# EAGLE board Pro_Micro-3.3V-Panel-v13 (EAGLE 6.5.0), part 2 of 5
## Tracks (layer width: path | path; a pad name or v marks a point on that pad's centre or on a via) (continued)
A16
  Top 0.203: U6.37 56.7,23.8 58.35,23.8 58.7,23.45 58.7,22.86 59.94,21.62 JP9.7
A17
  Top 0.203: U6.36 56.96,23.38 58.04,23.38 58.21,23.2 58.21,22.8 58.7,22.3 58.7,19.53 JP9.8
A20
  Top 0.203: 74.4,24.62 74.41,24.62 | 73.32,23.54 74.41,24.62 | 74.41,24.62 76.94,24.62 JP13.5
A21
  Top 0.203: U8.38 74.7,24.22 77.38,24.22 JP13.6
A22
  Top 0.203: U8.37 74.98,23.8 76.63,23.8 76.99,23.45 76.99,22.86 78.23,21.62 JP13.7
A23
  Top 0.203: U8.36 75.25,23.38 76.33,23.38 76.5,23.2 76.5,22.8 76.99,22.3 76.99,19.53 JP13.8
A26
  Top 0.203: 92.69,24.62 92.7,24.62 | 91.61,23.54 92.7,24.62 | 92.7,24.62 95.23,24.62 JP17.5
A27
  Top 0.203: U10.38 92.99,24.22 95.67,24.22 JP17.6
A28
  Top 0.203: U10.37 93.27,23.8 94.92,23.8 95.28,23.45 95.28,22.86 96.52,21.62 JP17.7
A29
  Top 0.203: U10.36 93.54,23.38 94.62,23.38 94.79,23.2 94.79,22.8 95.28,22.3 95.28,19.53 JP17.8
A32
  Top 0.203: 110.98,24.62 | 109.9,23.54 110.98,24.62 | 110.98,24.62 113.52,24.62 JP21.5
A33
  Top 0.203: U12.38 111.28,24.22 113.95,24.22 JP21.6
A34
  Top 0.203: U12.37 111.56,23.8 113.21,23.8 113.57,23.45 113.57,22.86 114.81,21.62 JP21.7
A35
  Top 0.203: U12.36 111.83,23.38 112.91,23.38 113.08,23.2 113.08,22.8 113.57,22.3 113.57,19.53 JP21.8
A38
  Top 0.203: 19.54,61.45 19.55,61.45 | 18.46,60.37 19.55,61.45 | 19.55,61.45 22.08,61.45 JP25.5
A39
  Top 0.203: U14.38 19.84,61.05 22.52,61.05 JP25.6
A40
  Top 0.203: U14.37 20.12,60.63 21.77,60.63 22.13,60.28 22.13,59.7 23.37,58.45 JP25.7
A41
  Top 0.203: U14.36 20.39,60.21 21.47,60.21 21.64,60.03 21.64,59.63 22.13,59.13 22.13,56.36 JP25.8
A44
  Top 0.203: 37.83,61.45 | 36.74,60.37 37.83,61.45 | 37.83,61.45 40.37,61.45 41.65,62.74 JP29.5
A45
  Top 0.203: U16.38 38.13,61.05 40.8,61.05 JP29.6
A46
  Top 0.203: U16.37 38.41,60.63 40.06,60.63 40.41,60.28 40.41,59.7 41.66,58.45 JP29.7
A47
  Top 0.203: U16.36 38.67,60.21 39.75,60.21 39.92,60.03 39.92,59.63 40.42,59.13 40.42,56.36 JP29.8
A50
  Top 0.203: 56.11,61.45 56.12,61.45 | 55.03,60.37 56.12,61.45 | 56.12,61.45 58.65,61.45 JP33.5
A51
  Top 0.203: U18.38 56.41,61.05 59.09,61.05 JP33.6
A52
  Top 0.203: U18.37 56.7,60.63 58.35,60.63 58.7,60.28 58.7,59.7 59.94,58.45 JP33.7
A53
  Top 0.203: U18.36 56.96,60.21 58.04,60.21 58.21,60.03 58.21,59.63 58.7,59.13 58.7,56.36 JP33.8
A56
  Top 0.203: 74.4,61.45 74.41,61.45 | 73.32,60.37 74.41,61.45 | 74.41,61.45 76.94,61.45 JP37.5
A57
  Top 0.203: U20.38 74.7,61.05 77.38,61.05 JP37.6
A58
  Top 0.203: U20.37 74.98,60.63 76.63,60.63 76.99,60.28 76.99,59.7 78.23,58.45 JP37.7
A59
  Top 0.203: U20.36 75.25,60.21 76.33,60.21 76.5,60.03 76.5,59.63 76.99,59.13 76.99,56.36 JP37.8
A62
  Top 0.203: 92.69,61.45 92.7,61.45 | 91.61,60.37 92.7,61.45 | 92.7,61.45 95.23,61.45 JP41.5
A63
  Top 0.203: U22.38 92.99,61.05 95.67,61.05 JP41.6
A64
  Top 0.203: U22.37 93.27,60.63 94.92,60.63 95.28,60.28 95.28,59.7 96.52,58.45 JP41.7
A65
  Top 0.203: U22.36 93.54,60.21 94.62,60.21 94.79,60.03 94.79,59.63 95.28,59.13 95.28,56.36 JP41.8
A68
  Top 0.203: 110.98,61.45 | 109.9,60.37 110.98,61.45 | 110.98,61.45 113.52,61.45 JP45.5
A69
  Top 0.203: U24.38 111.28,61.05 113.95,61.05 JP45.6
A70
  Top 0.203: U24.37 111.56,60.63 113.21,60.63 113.57,60.28 113.57,59.7 114.81,58.45 JP45.7
A71
  Top 0.203: U24.36 111.83,60.21 112.91,60.21 113.08,60.03 113.08,59.63 113.57,59.13 113.57,56.36 JP45.8
A74
  Top 0.203: 19.54,98.28 19.55,98.28 | 18.46,97.2 19.55,98.28 | 19.55,98.28 22.08,98.28 JP49.5
A75
  Top 0.203: U26.38 19.84,97.88 22.52,97.88 JP49.6
A76
  Top 0.203: U26.37 20.12,97.47 21.77,97.47 22.13,97.11 22.13,96.53 23.37,95.28 JP49.7
A77
  Top 0.203: U26.36 20.39,97.04 21.47,97.04 21.64,96.86 21.64,96.46 22.13,95.96 22.13,93.19 JP49.8
A80
  Top 0.203: 37.83,98.28 | 36.74,97.2 37.83,98.28 | 37.83,98.28 40.37,98.28 41.65,99.57 JP53.5
A81
  Top 0.203: U28.38 38.13,97.88 40.8,97.88 JP53.6
A82
  Top 0.203: U28.37 38.41,97.47 40.06,97.47 40.41,97.11 40.41,96.53 41.66,95.28 JP53.7
A83
  Top 0.203: U28.36 38.67,97.04 39.75,97.04 39.92,96.86 39.92,96.46 40.42,95.96 40.42,93.19 JP53.8
A86
  Top 0.203: 56.11,98.28 56.12,98.28 | 55.03,97.2 56.12,98.28 | 56.12,98.28 58.65,98.28 JP57.5
A87
  Top 0.203: U30.38 56.41,97.88 59.09,97.88 JP57.6
A88
  Top 0.203: U30.37 56.7,97.47 58.35,97.47 58.7,97.11 58.7,96.53 59.94,95.28 JP57.7
A89
  Top 0.203: U30.36 56.96,97.04 58.04,97.04 58.21,96.86 58.21,96.46 58.7,95.96 58.7,93.19 JP57.8
A92
  Top 0.203: 74.4,98.28 74.41,98.28 | 73.32,97.2 74.41,98.28 | 74.41,98.28 76.94,98.28 JP61.5
A93
  Top 0.203: U32.38 74.7,97.88 77.38,97.88 JP61.6
A94
  Top 0.203: U32.37 74.98,97.47 76.63,97.47 76.99,97.11 76.99,96.53 78.23,95.28 JP61.7
A95
  Top 0.203: U32.36 75.25,97.04 76.33,97.04 76.5,96.86 76.5,96.46 76.99,95.96 76.99,93.19 JP61.8
A98
  Top 0.203: 92.69,98.28 92.7,98.28 | 91.61,97.2 92.7,98.28 | 92.7,98.28 95.23,98.28 JP65.5
A99
  Top 0.203: U34.38 92.99,97.88 95.67,97.88 JP65.6
A100
  Top 0.203: U34.37 93.27,97.47 94.92,97.47 95.28,97.11 95.28,96.53 96.52,95.28 JP65.7
A101
  Top 0.203: U34.36 93.54,97.04 94.62,97.04 94.79,96.86 94.79,96.46 95.28,95.96 95.28,93.19 JP65.8
A104
  Top 0.203: 110.98,98.28 | 109.9,97.2 110.98,98.28 | 110.98,98.28 113.52,98.28 JP69.5
A105
  Top 0.203: U36.38 111.28,97.88 113.95,97.88 JP69.6
A106
  Top 0.203: U36.37 111.56,97.47 113.21,97.47 113.57,97.11 113.57,96.53 114.81,95.28 JP69.7
A107
  Top 0.203: U36.36 111.83,97.04 112.91,97.04 113.08,96.86 113.08,96.46 113.57,95.96 113.57,93.19 JP69.8
AREF
  Top 0.203: 17.41,24.58 18.24,25.41 C1.2
AREF1
  Top 0.203: 35.7,24.58 36.53,25.41 C11.2
AREF2
  Top 0.203: 53.99,24.58 54.82,25.41 C22.2
AREF3
  Top 0.203: 72.27,24.58 73.11,25.41 C31.2
AREF4
  Top 0.203: 90.56,24.58 91.4,25.41 C40.2
AREF5
  Top 0.203: 108.85,24.58 109.68,25.41 C49.2
AREF6
  Top 0.203: 17.41,61.41 18.24,62.24 C58.2
AREF7
  Top 0.203: 35.7,61.41 36.53,62.24 C67.2
AREF8
  Top 0.203: 53.99,61.41 54.82,62.24 C76.2
AREF9
  Top 0.203: 72.27,61.41 73.11,62.24 C85.2
AREF10
  Top 0.203: 90.56,61.41 91.4,62.24 C94.2
AREF11
  Top 0.203: 108.85,61.41 109.68,62.24 C103.2
AREF12
  Top 0.203: 17.41,98.24 18.24,99.08 C112.2
AREF13
  Top 0.203: 35.7,98.24 36.53,99.08 C121.2
AREF14
  Top 0.203: 53.99,98.24 54.82,99.08 C130.2
AREF15
  Top 0.203: 72.27,98.24 73.11,99.08 C139.2
AREF16
  Top 0.203: 90.56,98.24 91.4,99.08 C148.2
AREF17
  Top 0.203: 108.85,98.24 109.68,99.08 C157.2
D1  (via drill 0.25)
  Top 0.203: 37.09,18.47 38.4,17.16 39.23,17.16 39.98,16.41 39.98,9.35 40.26,9.06 v40.3,9.06
  Bottom 0.203: JP4.1 27.18,7.37 39.9,7.37 40.3,7.77 v40.3,9.06
D2  (via drill 0.25)
  Top 0.203: 13.74,17.42 13.56,17.25 13.56,16.57 v13.31,16.32
  Bottom 0.203: v13.31,16.32 14.48,17.49 14.48,18.29 11.68,21.08 11.68,23.55 11.09,24.14 10.13,24.14 9.79,24.49 9.79,27.08 10.3,27.58 11.01,27.58 11.68,28.25 11.68,30.62 11.68,30.63 11.11,31.21 9.91,31.21 9.41,30.7 9.41,27.9 8.13,26.62 JP7.8
D3  (via drill 0.25)
  Top 0.203: 13.39,17.77 12.88,17.26 v12.85,17.26
  Bottom 0.203: JP7.7 9.4,22.1 9.4,20.32 9.91,19.81 9.91,18.41 11.06,17.26 v12.85,17.26
D4  (via drill 0.25)
  Top 0.203: 17.41,17.07 18.46,16.03 v18.46,15.62
  Bottom 0.203: JP7.6 9.4,19.56 9.4,17.58 9.78,17.2 9.78,14.81 10.27,14.31 10.27,12.12 10.75,11.65 15.79,11.65 17.44,13.3 17.44,13.96 18.46,14.98 v18.46,15.62
D5  (via drill 0.25)
  Top 0.203: 19.5,19.17 20.13,18.53 v20.49,18.53
  Bottom 0.203: JP7.5 9.4,17.02 9.4,15.24 9.36,15.2 9.36,14.62 9.85,14.12 9.85,11.93 10.62,11.16 15.91,11.16 17.86,13.1 17.86,13.72 17.87,13.72 18.57,14.41 19.11,14.41 19.72,15.02 19.72,15.55 18.97,16.3 17.99,16.3 17.7,16.59 17.7,17.42 18.27,17.99 19.94,17.99 v20.49,18.53
D6  (via drill 0.25)
  Top 0.203: v18.41,17.14 18.41,17.45 v18.41,17.14 | U3.27 18.41,17.46 v18.41,17.14
  Bottom 0.203: v18.41,17.14 18.86,17.14 20.23,15.78 20.23,14.88 19.35,14.01 18.73,14.01 18.27,13.55 18.27,12.88 16.03,10.63 10.39,10.63 9.37,11.66 9.37,13.93 8.13,15.17 JP7.4
D7  (via drill 0.25)
  Top 0.203: JP7.3 9.4,14.48 9.4,20.14 v10.09,20.83 | v10.56,30.44 10.56,30.4 10.77,30.18 10.77,29.34 11.03,29.07 12.8,29.07 13.05,29.32 13.52,29.32 13.95,28.89 13.95,28.3 13.7,28.05 13.7,27.37 13.89,27.19 15.57,27.19 15.57,27.17 15.95,26.79 16.58,26.79 16.68,26.68 16.68,25.93 16.1,25.34 15.4,25.34 15.1,25.64 14.93,25.64 14.78,25.5 14.78,25.28 U3.1 14.79,25.28
  Bottom 0.203: v10.56,30.44 10.52,30.44 9.86,29.78 9.86,27.75 9.4,27.29 9.4,22.99 10.09,22.3 v10.09,20.83
D8  (via drill 0.25)
  Top 0.203: U3.28 19.84,16.74 20.66,16.74 21.23,16.16 21.23,9.53 21.25,9.51 v21.25,8.12
  Bottom 0.203: JP7.2 11,7.8 20.93,7.8 v21.25,8.12
D9  (via drill 0.25)
  Top 0.203: 18.8,18.47 20.12,17.16 20.94,17.16 21.69,16.41 21.69,9.35 21.97,9.06 v22.02,9.06
  Bottom 0.203: JP7.1 8.89,7.37 21.61,7.37 22.02,7.77 v22.02,9.06
D10
  Top 0.203: JP6.12 23.37,8.81 22.12,10.06 22.12,16.56 21.1,17.58 20.39,17.58 U3.30
D14  (via drill 0.25)
  Top 0.203: R4.1 9.65,9.56 9.65,11.68 9.81,11.84 9.81,18.19 v10.57,18.96 | 12.35,22.83 11.81,23.37 v10.92,23.37
  Bottom 0.203: v10.92,23.37 10.92,19.31 v10.57,18.96
D15  (via drill 0.25)
  Top 0.203: U4.28 38.13,16.74 38.95,16.74 39.52,16.16 39.52,9.53 39.53,9.51 v39.53,8.12
  Bottom 0.203: JP4.2 29.29,7.8 39.22,7.8 v39.53,8.12
D16  (via drill 0.25)
  Top 0.203: 32.02,17.42 31.85,17.25 31.85,16.57 v31.59,16.32
  Bottom 0.203: v31.59,16.32 32.77,17.49 32.77,18.29 29.97,21.08 29.97,23.55 29.38,24.14 28.42,24.14 28.08,24.49 28.08,27.08 28.59,27.58 29.3,27.58 29.97,28.25 29.97,30.62 29.97,30.63 29.39,31.21 28.2,31.21 27.7,30.7 27.7,27.9 26.42,26.62 JP4.8
D17  (via drill 0.25)
  Top 0.203: 31.68,17.77 31.17,17.26 v31.14,17.26
  Bottom 0.203: JP4.7 27.69,22.1 27.69,20.32 28.19,19.81 28.19,18.41 29.34,17.26 v31.14,17.26
D18  (via drill 0.25)
  Top 0.203: 35.7,17.07 36.74,16.03 v36.74,15.62
  Bottom 0.203: JP4.6 27.69,19.56 27.69,17.58 28.07,17.2 28.07,14.81 28.56,14.31 28.56,12.12 29.04,11.65 34.07,11.65 35.73,13.3 35.73,13.96 36.74,14.98 v36.74,15.62
D19  (via drill 0.25)
  Top 0.203: 37.79,19.17 38.42,18.53 v38.78,18.53
  Bottom 0.203: JP4.5 27.69,17.02 27.69,15.24 27.64,15.2 27.64,14.62 28.14,14.12 28.14,11.93 28.91,11.16 34.2,11.16 36.14,13.1 36.14,13.72 36.16,13.72 36.85,14.41 37.4,14.41 38.01,15.02 38.01,15.55 37.26,16.3 36.28,16.3 35.99,16.59 35.99,17.42 36.56,17.99 38.23,17.99 v38.78,18.53
D20  (via drill 0.25)
  Top 0.203: v36.7,17.14 36.7,17.45 v36.7,17.14 | U4.27 36.7,17.46 v36.7,17.14
  Bottom 0.203: v36.7,17.14 37.15,17.14 38.52,15.78 38.52,14.88 37.64,14.01 37.02,14.01 36.56,13.55 36.56,12.88 34.31,10.63 28.68,10.63 27.66,11.66 27.66,13.93 26.42,15.17 JP4.4
D21  (via drill 0.25)
  Top 0.203: JP4.3 27.69,14.48 27.69,20.14 v28.38,20.83 | v28.84,30.44 28.84,30.4 29.06,30.18 29.06,29.34 29.32,29.07 31.09,29.07 31.34,29.32 31.81,29.32 32.23,28.89 32.23,28.3 31.99,28.05 31.99,27.37 32.17,27.19 33.86,27.19 33.86,27.17 34.24,26.79 34.86,26.79 34.97,26.68 34.97,25.93 34.38,25.34 33.69,25.34 33.39,25.64 33.21,25.64 33.07,25.5 33.07,25.28 U4.1 33.07,25.28
  Bottom 0.203: v28.84,30.44 28.81,30.44 28.14,29.78 28.14,27.75 27.69,27.29 27.69,22.99 28.38,22.3 v28.38,20.83
D22
  Top 0.203: JP3.12 41.66,8.81 40.41,10.06 40.41,16.56 39.38,17.58 38.67,17.58 U4.30
D26  (via drill 0.25)
  Top 0.203: R9.1 27.94,9.56 27.94,11.68 28.09,11.84 28.09,18.19 v28.86,18.96 | 30.64,22.83 30.1,23.37 v29.21,23.37
  Bottom 0.203: v29.21,23.37 29.21,19.31 v28.86,18.96
D27  (via drill 0.25)
  Top 0.203: 55.38,18.47 56.69,17.16 57.52,17.16 58.27,16.41 58.27,9.35 58.55,9.06 v58.59,9.06
  Bottom 0.203: JP10.1 45.47,7.37 58.19,7.37 58.59,7.77 v58.59,9.06
D28  (via drill 0.25)
  Top 0.203: U6.28 56.42,16.74 57.24,16.74 57.81,16.16 57.81,9.53 57.82,9.51 v57.82,8.12
  Bottom 0.203: JP10.2 47.57,7.8 57.5,7.8 v57.82,8.12
D29  (via drill 0.25)
  Top 0.203: 50.31,17.42 50.14,17.25 50.14,16.57 v49.88,16.32
  Bottom 0.203: v49.88,16.32 51.05,17.49 51.05,18.29 48.26,21.08 48.26,23.55 47.67,24.14 46.71,24.14 46.37,24.49 46.37,27.08 46.88,27.58 47.59,27.58 48.26,28.25 48.26,30.62 48.26,30.63 47.68,31.21 46.49,31.21 45.99,30.7 45.99,27.9 44.7,26.62 JP10.8
D30  (via drill 0.25)
  Top 0.203: 49.97,17.77 49.96,17.77 49.46,17.26 v49.42,17.26
  Bottom 0.203: JP10.7 45.97,22.1 45.97,20.32 46.48,19.81 46.48,18.41 47.63,17.26 v49.42,17.26
D31  (via drill 0.25)
  Top 0.203: 53.99,17.07 55.03,16.03 v55.03,15.62
  Bottom 0.203: JP10.6 45.97,19.56 45.97,17.58 46.35,17.2 46.35,14.81 46.85,14.31 46.85,12.12 47.33,11.65 52.36,11.65 54.02,13.3 54.02,13.96 55.03,14.98 v55.03,15.62
D32  (via drill 0.25)
  Top 0.203: 56.08,19.17 56.71,18.53 v57.06,18.53
  Bottom 0.203: JP10.5 45.97,17.02 45.97,15.24 45.93,15.2 45.93,14.62 46.43,14.12 46.43,11.93 47.19,11.16 52.49,11.16 54.43,13.1 54.43,13.72 54.45,13.72 55.14,14.41 55.68,14.41 56.29,15.02 56.29,15.55 55.55,16.3 54.56,16.3 54.28,16.59 54.28,17.42 54.85,17.99 56.52,17.99 v57.06,18.53
D33  (via drill 0.25)
  Top 0.203: v54.99,17.14 54.99,17.45 v54.99,17.14 | U6.27 54.99,17.46 v54.99,17.14
  Bottom 0.203: v54.99,17.14 55.44,17.14 56.81,15.78 56.81,14.88 55.93,14.01 55.31,14.01 54.85,13.55 54.85,12.88 52.6,10.63 46.97,10.63 45.95,11.66 45.95,13.93 44.7,15.17 JP10.4
D34  (via drill 0.25)
  Top 0.203: JP10.3 45.97,14.48 45.97,20.14 v46.66,20.83 | v47.13,30.44 47.13,30.4 47.35,30.18 47.35,29.34 47.61,29.07 49.38,29.07 49.63,29.32 50.09,29.32 50.52,28.89 50.52,28.3 50.28,28.05 50.28,27.37 50.46,27.19 52.15,27.19 52.15,27.17 52.53,26.79 53.15,26.79 53.25,26.68 53.25,25.93 52.67,25.34 51.98,25.34 51.68,25.64 51.5,25.64 51.35,25.5 51.35,25.28 U6.1 51.36,25.28
  Bottom 0.203: v47.13,30.44 47.1,30.44 46.43,29.78 46.43,27.75 45.97,27.29 45.97,22.99 46.66,22.3 v46.66,20.83
D35
  Top 0.203: JP9.12 59.94,8.81 58.7,10.06 58.7,16.56 57.67,17.58 56.96,17.58 U6.30
D39  (via drill 0.25)
  Top 0.203: R16.1 46.23,9.56 46.23,11.68 46.38,11.84 46.38,18.19 v47.15,18.96 | 48.93,22.83 48.39,23.37 v47.5,23.37
  Bottom 0.203: v47.5,23.37 47.5,19.31 v47.15,18.96
D40  (via drill 0.25)
  Top 0.203: 73.67,18.47 74.98,17.16 75.81,17.16 76.56,16.41 76.56,9.35 76.84,9.06 v76.88,9.06
  Bottom 0.203: JP14.1 63.75,7.37 76.48,7.37 76.88,7.77 v76.88,9.06
D41  (via drill 0.25)
  Top 0.203: U8.28 74.7,16.74 75.53,16.74 76.1,16.16 76.1,9.53 76.11,9.51 v76.11,8.12
  Bottom 0.203: JP14.2 65.86,7.8 75.79,7.8 v76.11,8.12
D42  (via drill 0.25)
  Top 0.203: 68.6,17.42 68.43,17.25 68.43,16.57 v68.17,16.32
  Bottom 0.203: v68.17,16.32 69.34,17.49 69.34,18.29 66.55,21.08 66.55,23.55 65.96,24.14 65,24.14 64.66,24.49 64.66,27.08 65.16,27.58 65.88,27.58 66.55,28.25 66.55,30.62 66.55,30.63 65.97,31.21 64.78,31.21 64.28,30.7 64.28,27.9 62.99,26.62 JP14.8
D43  (via drill 0.25)
  Top 0.203: 68.25,17.77 67.74,17.26 v67.71,17.26
  Bottom 0.203: JP14.7 64.26,22.1 64.26,20.32 64.77,19.81 64.77,18.41 65.92,17.26 v67.71,17.26
D44  (via drill 0.25)
  Top 0.203: 72.27,17.07 73.32,16.03 v73.32,15.62
  Bottom 0.203: JP14.6 64.26,19.56 64.26,17.58 64.64,17.2 64.64,14.81 65.14,14.31 65.14,12.12 65.61,11.65 70.65,11.65 72.31,13.3 72.31,13.96 73.32,14.98 v73.32,15.62
D45  (via drill 0.25)
  Top 0.203: 74.37,19.17 75,18.53 v75.35,18.53
  Bottom 0.203: JP14.5 64.26,17.02 64.26,15.24 64.22,15.2 64.22,14.62 64.72,14.12 64.72,11.93 65.48,11.16 70.78,11.16 72.72,13.1 72.72,13.72 72.73,13.72 73.43,14.41 73.97,14.41 74.58,15.02 74.58,15.55 73.83,16.3 72.85,16.3 72.57,16.59 72.57,17.42 73.13,17.99 74.81,17.99 v75.35,18.53
D46  (via drill 0.25)
  Top 0.203: v73.28,17.14 73.28,17.45 v73.28,17.14 | U8.27 73.28,17.46 v73.28,17.14
  Bottom 0.203: v73.28,17.14 73.73,17.14 75.09,15.78 75.09,14.88 74.22,14.01 73.59,14.01 73.13,13.55 73.13,12.88 70.89,10.63 65.25,10.63 64.23,11.66 64.23,13.93 62.99,15.17 JP14.4
D47  (via drill 0.25)
  Top 0.203: JP14.3 64.26,14.48 64.26,20.14 v64.95,20.83 | v65.42,30.44 65.42,30.4 65.63,30.18 65.63,29.34 65.89,29.07 67.67,29.07 67.92,29.32 68.38,29.32 68.81,28.89 68.81,28.3 68.57,28.05 68.57,27.37 68.75,27.19 70.44,27.19 70.44,27.17 70.82,26.79 71.44,26.79 71.54,26.68 71.54,25.93 70.96,25.34 70.27,25.34 69.97,25.64 69.79,25.64 69.64,25.5 69.64,25.28 U8.1 69.65,25.28
  Bottom 0.203: v65.42,30.44 65.39,30.44 64.72,29.78 64.72,27.75 64.26,27.29 64.26,22.99 64.95,22.3 v64.95,20.83
D48
  Top 0.203: JP13.12 78.23,8.81 76.99,10.06 76.99,16.56 75.96,17.58 75.25,17.58 U8.30
D52  (via drill 0.25)
  Top 0.203: R22.1 64.52,9.56 64.52,11.68 64.67,11.84 64.67,18.19 v65.44,18.96 | 67.22,22.83 66.68,23.37 v65.79,23.37
  Bottom 0.203: v65.79,23.37 65.79,19.31 v65.44,18.96
D53  (via drill 0.25)
  Top 0.203: 91.96,18.47 93.27,17.16 94.09,17.16 94.84,16.41 94.84,9.35 95.13,9.06 v95.17,9.06
  Bottom 0.203: JP18.1 82.04,7.37 94.77,7.37 95.17,7.77 v95.17,9.06
D54  (via drill 0.25)
  Top 0.203: U10.28 92.99,16.74 93.81,16.74 94.39,16.16 94.39,9.53 94.4,9.51 v94.4,8.12
  Bottom 0.203: JP18.2 84.15,7.8 94.08,7.8 v94.4,8.12
D55  (via drill 0.25)
  Top 0.203: 86.89,17.42 86.72,17.25 86.72,16.57 v86.46,16.32
  Bottom 0.203: v86.46,16.32 87.63,17.49 87.63,18.29 84.84,21.08 84.84,23.55 84.24,24.14 83.29,24.14 82.94,24.49 82.94,27.08 83.45,27.58 84.16,27.58 84.83,28.25 84.83,30.62 84.84,30.63 84.26,31.21 83.07,31.21 82.56,30.7 82.56,27.9 81.28,26.62 JP18.8
D56  (via drill 0.25)
  Top 0.203: 86.54,17.77 86.03,17.26 v86,17.26
  Bottom 0.203: JP18.7 82.55,22.1 82.55,20.32 83.06,19.81 83.06,18.41 84.21,17.26 v86,17.26
D57  (via drill 0.25)
  Top 0.203: 90.56,17.07 91.61,16.03 v91.61,15.62
  Bottom 0.203: JP18.6 82.55,19.56 82.55,17.58 82.93,17.2 82.93,14.81 83.43,14.31 83.43,12.12 83.9,11.65 88.94,11.65 90.59,13.3 90.59,13.96 91.61,14.98 v91.61,15.62
D58  (via drill 0.25)
  Top 0.203: 92.65,19.17 93.28,18.53 v93.64,18.53
  Bottom 0.203: JP18.5 82.55,17.02 82.55,15.24 82.51,15.2 82.51,14.62 83,14.12 83,11.93 83.77,11.16 89.06,11.16 91.01,13.1 91.01,13.72 91.02,13.72 91.72,14.41 92.26,14.41 92.87,15.02 92.87,15.55 92.12,16.3 91.14,16.3 90.86,16.59 90.86,17.42 91.42,17.99 93.1,17.99 v93.64,18.53
D59  (via drill 0.25)
  Top 0.203: v91.57,17.14 91.57,17.45 v91.57,17.14 | U10.27 91.57,17.46 v91.57,17.14
  Bottom 0.203: v91.57,17.14 92.02,17.14 93.38,15.78 93.38,14.88 92.5,14.01 91.88,14.01 91.42,13.55 91.42,12.88 89.18,10.63 83.54,10.63 82.52,11.66 82.52,13.93 81.28,15.17 JP18.4
D60  (via drill 0.25)
  Top 0.203: JP18.3 82.55,14.48 82.55,20.14 v83.24,20.83 | v83.71,30.44 83.71,30.4 83.92,30.18 83.92,29.34 84.18,29.07 85.96,29.07 86.2,29.32 86.67,29.32 87.1,28.89 87.1,28.3 86.86,28.05 86.86,27.37 87.04,27.19 88.72,27.19 88.72,27.17 89.11,26.79 89.73,26.79 89.83,26.68 89.83,25.93 89.25,25.34 88.56,25.34 88.25,25.64 88.08,25.64 87.93,25.5 87.93,25.28 U10.1 87.94,25.28
  Bottom 0.203: v83.71,30.44 83.67,30.44 83.01,29.78 83.01,27.75 82.55,27.29 82.55,22.99 83.24,22.3 v83.24,20.83
D61
  Top 0.203: JP17.12 96.52,8.81 95.28,10.06 95.28,16.56 94.25,17.58 93.54,17.58 U10.30
D65  (via drill 0.25)
  Top 0.203: R28.1 82.8,9.56 82.8,11.68 82.96,11.84 82.96,18.19 v83.73,18.96 | 85.51,22.83 84.97,23.37 v84.07,23.37
  Bottom 0.203: v84.07,23.37 84.07,19.31 v83.73,18.96
D66  (via drill 0.25)
  Top 0.203: 110.24,18.47 111.56,17.16 112.38,17.16 113.13,16.41 113.13,9.35 113.41,9.06 v113.46,9.06
  Bottom 0.203: JP22.1 100.33,7.37 113.06,7.37 113.46,7.77 v113.46,9.06
D67  (via drill 0.25)
  Top 0.203: U12.28 111.28,16.74 112.1,16.74 112.67,16.16 112.67,9.53 112.69,9.51 v112.69,8.12
  Bottom 0.203: JP22.2 102.44,7.8 112.37,7.8 v112.69,8.12
D68  (via drill 0.25)
  Top 0.203: 105.18,17.42 105,17.25 105,16.57 v104.75,16.32
  Bottom 0.203: v104.75,16.32 105.92,17.49 105.92,18.29 103.12,21.08 103.12,23.55 102.53,24.14 101.58,24.14 101.23,24.49 101.23,27.08 101.74,27.58 102.45,27.58 103.12,28.25 103.12,30.62 103.12,30.63 102.55,31.21 101.35,31.21 100.85,30.7 100.85,27.9 99.57,26.62 JP22.8
D69  (via drill 0.25)
  Top 0.203: 104.83,17.77 104.32,17.26 v104.29,17.26
  Bottom 0.203: JP22.7 100.84,22.1 100.84,20.32 101.35,19.81 101.35,18.41 102.5,17.26 v104.29,17.26
D70  (via drill 0.25)
  Top 0.203: 108.85,17.07 109.9,16.03 v109.9,15.62
  Bottom 0.203: JP22.6 100.84,19.56 100.84,17.58 101.22,17.2 101.22,14.81 101.71,14.31 101.71,12.12 102.19,11.65 107.23,11.65 108.88,13.3 108.88,13.96 109.9,14.98 v109.9,15.62
D71  (via drill 0.25)
  Top 0.203: 110.94,19.17 111.57,18.53 v111.93,18.53
  Bottom 0.203: JP22.5 100.84,17.02 100.84,15.24 100.8,15.2 100.8,14.62 101.29,14.12 101.29,11.93 102.06,11.16 107.35,11.16 109.3,13.1 109.3,13.72 109.31,13.72 110,14.41 110.55,14.41 111.16,15.02 111.16,15.55 110.41,16.3 109.43,16.3 109.14,16.59 109.14,17.42 109.71,17.99 111.38,17.99 v111.93,18.53
D72  (via drill 0.25)
  Top 0.203: v109.86,17.14 109.86,17.45 v109.86,17.14 | U12.27 109.86,17.46 v109.86,17.14
  Bottom 0.203: v109.86,17.14 110.31,17.14 111.67,15.78 111.67,14.88 110.79,14.01 110.17,14.01 109.71,13.55 109.71,12.88 107.47,10.63 101.83,10.63 100.81,11.66 100.81,13.93 99.57,15.17 JP22.4
D73  (via drill 0.25)
  Top 0.203: JP22.3 100.84,14.48 100.84,20.14 v101.53,20.83 | v102,30.44 102,30.4 102.21,30.18 102.21,29.34 102.47,29.07 104.24,29.07 104.49,29.32 104.96,29.32 105.39,28.89 105.39,28.3 105.14,28.05 105.14,27.37 105.33,27.19 107.01,27.19 107.01,27.17 107.39,26.79 108.02,26.79 108.12,26.68 108.12,25.93 107.54,25.34 106.84,25.34 106.54,25.64 106.36,25.64 106.22,25.5 106.22,25.28 U12.1 106.22,25.28
  Bottom 0.203: v102,30.44 101.96,30.44 101.3,29.78 101.3,27.75 100.84,27.29 100.84,22.99 101.53,22.3 v101.53,20.83
D74
  Top 0.203: JP21.12 114.81,8.81 113.56,10.06 113.56,16.56 112.54,17.58 111.83,17.58 U12.30
D78  (via drill 0.25)
  Top 0.203: R34.1 101.09,9.56 101.09,11.68 101.25,11.84 101.25,18.19 v102.01,18.96 | 103.79,22.83 103.25,23.37 v102.36,23.37
  Bottom 0.203: v102.36,23.37 102.36,19.31 v102.01,18.96
D79  (via drill 0.25)
  Top 0.203: 18.8,55.3 20.12,53.99 20.94,53.99 21.69,53.24 21.69,46.18 21.97,45.9 v22.02,45.9
  Bottom 0.203: JP26.1 8.89,44.2 21.61,44.2 22.02,44.6 v22.02,45.9
D80  (via drill 0.25)
  Top 0.203: U14.28 19.84,53.57 20.66,53.57 21.23,52.99 21.23,46.35 21.25,46.34 v21.25,44.95
  Bottom 0.203: JP26.2 11,44.63 20.93,44.63 v21.25,44.95
D81  (via drill 0.25)
  Top 0.203: 13.74,54.25 13.56,54.08 13.56,53.4 v13.31,53.15
  Bottom 0.203: v13.31,53.15 14.48,54.32 14.48,55.12 11.68,57.91 11.68,60.38 11.09,60.97 10.13,60.97 9.79,61.32 9.79,63.91 10.3,64.41 11.01,64.41 11.68,65.08 11.68,67.45 11.68,67.46 11.11,68.04 9.91,68.04 9.41,67.53 9.41,64.73 8.13,63.45 JP26.8
D82  (via drill 0.25)
  Top 0.203: 13.39,54.6 12.88,54.09 v12.85,54.09
  Bottom 0.203: JP26.7 9.4,58.93 9.4,57.15 9.91,56.64 9.91,55.24 11.06,54.09 v12.85,54.09
D83  (via drill 0.25)
  Top 0.203: 17.41,53.9 18.46,52.86 v18.46,52.45
  Bottom 0.203: JP26.6 9.4,56.39 9.4,54.41 9.78,54.03 9.78,51.64 10.27,51.14 10.27,48.95 10.75,48.48 15.79,48.48 17.44,50.13 17.44,50.79 18.46,51.81 v18.46,52.45
D84  (via drill 0.25)
  Top 0.203: 19.5,56 20.13,55.36 v20.49,55.36
  Bottom 0.203: JP26.5 9.4,53.85 9.4,52.07 9.36,52.03 9.36,51.45 9.85,50.95 9.85,48.76 10.62,47.99 15.91,47.99 17.86,49.93 17.86,50.55 17.87,50.55 18.57,51.24 19.11,51.24 19.72,51.85 19.72,52.38 18.97,53.13 17.99,53.13 17.7,53.42 17.7,54.25 18.27,54.82 19.94,54.82 v20.49,55.36
D85  (via drill 0.25)
  Top 0.203: v18.41,53.98 18.41,54.28 v18.41,53.98 | U14.27 18.41,54.29 v18.41,53.98
  Bottom 0.203: v18.41,53.98 18.86,53.98 20.23,52.61 20.23,51.71 19.35,50.84 18.73,50.84 18.27,50.38 18.27,49.71 16.03,47.47 10.39,47.47 9.37,48.49 9.37,50.76 8.13,52 JP26.4
D86  (via drill 0.25)
  Top 0.203: JP26.3 9.4,51.31 9.4,56.97 v10.09,57.66 | v10.56,67.27 10.56,67.23 10.77,67.01 10.77,66.17 11.03,65.91 12.8,65.91 13.05,66.15 13.52,66.15 13.95,65.72 13.95,65.13 13.7,64.88 13.7,64.2 13.89,64.02 15.57,64.02 15.57,64 15.95,63.62 16.58,63.62 16.68,63.52 16.68,62.76 16.1,62.17 15.4,62.17 15.1,62.47 14.93,62.47 14.78,62.33 14.78,62.11 U14.1 14.79,62.11
  Bottom 0.203: v10.56,67.27 10.52,67.27 9.86,66.61 9.86,64.58 9.4,64.12 9.4,59.82 10.09,59.13 v10.09,57.66
D87
  Top 0.203: JP25.12 23.37,45.64 22.12,46.89 22.12,53.39 21.1,54.41 20.39,54.41 U14.30
D91  (via drill 0.25)
  Top 0.203: R40.1 9.65,46.39 9.65,48.51 9.81,48.67 9.81,55.02 v10.57,55.79 | 12.35,59.66 11.81,60.2 v10.92,60.2
  Bottom 0.203: v10.92,60.2 10.92,56.14 v10.57,55.79
D92  (via drill 0.25)
  Top 0.203: 37.09,55.3 38.4,53.99 39.23,53.99 39.98,53.24 39.98,46.18 40.26,45.9 v40.3,45.9
  Bottom 0.203: JP30.1 27.18,44.2 39.9,44.2 40.3,44.6 v40.3,45.9
D93  (via drill 0.25)
  Top 0.203: U16.28 38.13,53.57 38.95,53.57 39.52,52.99 39.52,46.35 39.53,46.34 v39.53,44.95
  Bottom 0.203: JP30.2 29.29,44.63 39.22,44.63 v39.53,44.95
D94  (via drill 0.25)
  Top 0.203: 32.02,54.25 31.85,54.08 31.85,53.4 v31.59,53.15
  Bottom 0.203: v31.59,53.15 32.77,54.32 32.77,55.12 29.97,57.91 29.97,60.38 29.38,60.97 28.42,60.97 28.08,61.32 28.08,63.91 28.59,64.41 29.3,64.41 29.97,65.08 29.97,67.45 29.97,67.46 29.39,68.04 28.2,68.04 27.7,67.53 27.7,64.73 26.42,63.45 JP30.8
D95  (via drill 0.25)
  Top 0.203: 31.68,54.6 31.17,54.09 v31.14,54.09
  Bottom 0.203: JP30.7 27.69,58.93 27.69,57.15 28.19,56.64 28.19,55.24 29.34,54.09 v31.14,54.09
D96  (via drill 0.25)
  Top 0.203: 35.7,53.9 36.74,52.86 v36.74,52.45
  Bottom 0.203: JP30.6 27.69,56.39 27.69,54.41 28.07,54.03 28.07,51.64 28.56,51.14 28.56,48.95 29.04,48.48 34.07,48.48 35.73,50.13 35.73,50.79 36.74,51.81 v36.74,52.45
D97  (via drill 0.25)
  Top 0.203: 37.79,56 38.42,55.36 v38.78,55.36
  Bottom 0.203: JP30.5 27.69,53.85 27.69,52.07 27.64,52.03 27.64,51.45 28.14,50.95 28.14,48.76 28.91,47.99 34.2,47.99 36.14,49.93 36.14,50.55 36.16,50.55 36.85,51.24 37.4,51.24 38.01,51.85 38.01,52.38 37.26,53.13 36.28,53.13 35.99,53.42 35.99,54.25 36.56,54.82 38.23,54.82 v38.78,55.36
D98  (via drill 0.25)
  Top 0.203: v36.7,53.98 36.7,54.28 v36.7,53.98 | U16.27 36.7,54.29 v36.7,53.98
  Bottom 0.203: v36.7,53.98 37.15,53.98 38.52,52.61 38.52,51.71 37.64,50.84 37.02,50.84 36.56,50.38 36.56,49.71 34.31,47.47 28.68,47.47 27.66,48.49 27.66,50.76 26.42,52 JP30.4
D99  (via drill 0.25)
  Top 0.203: JP30.3 27.69,51.31 27.69,56.97 v28.38,57.66 | v28.84,67.27 28.84,67.23 29.06,67.01 29.06,66.17 29.32,65.91 31.09,65.91 31.34,66.15 31.81,66.15 32.23,65.72 32.23,65.13 31.99,64.88 31.99,64.2 32.17,64.02 33.86,64.02 33.86,64 34.24,63.62 34.86,63.62 34.97,63.52 34.97,62.76 34.38,62.17 33.69,62.17 33.39,62.47 33.21,62.47 33.07,62.33 33.07,62.11 U16.1 33.07,62.11
  Bottom 0.203: v28.84,67.27 28.81,67.27 28.14,66.61 28.14,64.58 27.69,64.12 27.69,59.82 28.38,59.13 v28.38,57.66
D100
  Top 0.203: JP29.12 41.66,45.64 40.41,46.89 40.41,53.39 39.38,54.41 38.67,54.41 U16.30
D104  (via drill 0.25)
  Top 0.203: R46.1 27.94,46.39 27.94,48.51 28.09,48.67 28.09,55.02 v28.86,55.79 | 30.64,59.66 30.1,60.2 v29.21,60.2
  Bottom 0.203: v29.21,60.2 29.21,56.14 v28.86,55.79
D105  (via drill 0.25)
  Top 0.203: 55.38,55.3 56.69,53.99 57.52,53.99 58.27,53.24 58.27,46.18 58.55,45.9 v58.59,45.9
  Bottom 0.203: JP34.1 45.47,44.2 58.19,44.2 58.59,44.6 v58.59,45.9
D106  (via drill 0.25)
  Top 0.203: U18.28 56.42,53.57 57.24,53.57 57.81,52.99 57.81,46.35 57.82,46.34 v57.82,44.95
  Bottom 0.203: JP34.2 47.57,44.63 57.5,44.63 v57.82,44.95
D107  (via drill 0.25)
  Top 0.203: 50.31,54.25 50.14,54.08 50.14,53.4 v49.88,53.15
  Bottom 0.203: v49.88,53.15 51.05,54.32 51.05,55.12 48.26,57.91 48.26,60.38 47.67,60.97 46.71,60.97 46.37,61.32 46.37,63.91 46.88,64.41 47.59,64.41 48.26,65.08 48.26,67.45 48.26,67.46 47.68,68.04 46.49,68.04 45.99,67.53 45.99,64.73 44.7,63.45 JP34.8
D108  (via drill 0.25)
  Top 0.203: 49.97,54.6 49.96,54.6 49.46,54.09 v49.42,54.09
  Bottom 0.203: JP34.7 45.97,58.93 45.97,57.15 46.48,56.64 46.48,55.24 47.63,54.09 v49.42,54.09
D109  (via drill 0.25)
  Top 0.203: 53.99,53.9 55.03,52.86 v55.03,52.45
  Bottom 0.203: JP34.6 45.97,56.39 45.97,54.41 46.35,54.03 46.35,51.64 46.85,51.14 46.85,48.95 47.33,48.48 52.36,48.48 54.02,50.13 54.02,50.79 55.03,51.81 v55.03,52.45
D110  (via drill 0.25)
  Top 0.203: 56.08,56 56.71,55.36 v57.06,55.36
  Bottom 0.203: JP34.5 45.97,53.85 45.97,52.07 45.93,52.03 45.93,51.45 46.43,50.95 46.43,48.76 47.19,47.99 52.49,47.99 54.43,49.93 54.43,50.55 54.45,50.55 55.14,51.24 55.68,51.24 56.29,51.85 56.29,52.38 55.55,53.13 54.56,53.13 54.28,53.42 54.28,54.25 54.85,54.82 56.52,54.82 v57.06,55.36
D111  (via drill 0.25)
  Top 0.203: v54.99,53.98 54.99,54.28 v54.99,53.98 | U18.27 54.99,54.29 v54.99,53.98
  Bottom 0.203: v54.99,53.98 55.44,53.98 56.81,52.61 56.81,51.71 55.93,50.84 55.31,50.84 54.85,50.38 54.85,49.71 52.6,47.47 46.97,47.47 45.95,48.49 45.95,50.76 44.7,52 JP34.4
D112  (via drill 0.25)
  Top 0.203: JP34.3 45.97,51.31 45.97,56.97 v46.66,57.66 | v47.13,67.27 47.13,67.23 47.35,67.01 47.35,66.17 47.61,65.91 49.38,65.91 49.63,66.15 50.09,66.15 50.52,65.72 50.52,65.13 50.28,64.88 50.28,64.2 50.46,64.02 52.15,64.02 52.15,64 52.53,63.62 53.15,63.62 53.25,63.52 53.25,62.76 52.67,62.17 51.98,62.17 51.68,62.47 51.5,62.47 51.35,62.33 51.35,62.11 U18.1 51.36,62.11
  Bottom 0.203: v47.13,67.27 47.1,67.27 46.43,66.61 46.43,64.58 45.97,64.12 45.97,59.82 46.66,59.13 v46.66,57.66
D113
  Top 0.203: JP33.12 59.94,45.64 58.7,46.89 58.7,53.39 57.67,54.41 56.96,54.41 U18.30
D117  (via drill 0.25)
  Top 0.203: R52.1 46.23,46.39 46.23,48.51 46.38,48.67 46.38,55.02 v47.15,55.79 | 48.93,59.66 48.39,60.2 v47.5,60.2
  Bottom 0.203: v47.5,60.2 47.5,56.14 v47.15,55.79
D118  (via drill 0.25)
  Top 0.203: 73.67,55.3 74.98,53.99 75.81,53.99 76.56,53.24 76.56,46.18 76.84,45.9 v76.88,45.9
  Bottom 0.203: JP38.1 63.75,44.2 76.48,44.2 76.88,44.6 v76.88,45.9
D119  (via drill 0.25)
  Top 0.203: U20.28 74.7,53.57 75.53,53.57 76.1,52.99 76.1,46.35 76.11,46.34 v76.11,44.95
  Bottom 0.203: JP38.2 65.86,44.63 75.79,44.63 v76.11,44.95
D120  (via drill 0.25)
  Top 0.203: 68.6,54.25 68.43,54.08 68.43,53.4 v68.17,53.15
  Bottom 0.203: v68.17,53.15 69.34,54.32 69.34,55.12 66.55,57.91 66.55,60.38 65.96,60.97 65,60.97 64.66,61.32 64.66,63.91 65.16,64.41 65.88,64.41 66.55,65.08 66.55,67.45 66.55,67.46 65.97,68.04 64.78,68.04 64.28,67.53 64.28,64.73 62.99,63.45 JP38.8
D121  (via drill 0.25)
  Top 0.203: 68.25,54.6 67.74,54.09 v67.71,54.09
  Bottom 0.203: JP38.7 64.26,58.93 64.26,57.15 64.77,56.64 64.77,55.24 65.92,54.09 v67.71,54.09
D122  (via drill 0.25)
  Top 0.203: 72.27,53.9 73.32,52.86 v73.32,52.45
  Bottom 0.203: JP38.6 64.26,56.39 64.26,54.41 64.64,54.03 64.64,51.64 65.14,51.14 65.14,48.95 65.61,48.48 70.65,48.48 72.31,50.13 72.31,50.79 73.32,51.81 v73.32,52.45
D123  (via drill 0.25)
  Top 0.203: 74.37,56 75,55.36 v75.35,55.36
  Bottom 0.203: JP38.5 64.26,53.85 64.26,52.07 64.22,52.03 64.22,51.45 64.72,50.95 64.72,48.76 65.48,47.99 70.78,47.99 72.72,49.93 72.72,50.55 72.73,50.55 73.43,51.24 73.97,51.24 74.58,51.85 74.58,52.38 73.83,53.13 72.85,53.13 72.57,53.42 72.57,54.25 73.13,54.82 74.81,54.82 v75.35,55.36
D124  (via drill 0.25)
  Top 0.203: v73.28,53.98 73.28,54.28 v73.28,53.98 | U20.27 73.28,54.29 v73.28,53.98
  Bottom 0.203: v73.28,53.98 73.73,53.98 75.09,52.61 75.09,51.71 74.22,50.84 73.59,50.84 73.13,50.38 73.13,49.71 70.89,47.47 65.25,47.47 64.23,48.49 64.23,50.76 62.99,52 JP38.4
D125  (via drill 0.25)
  Top 0.203: JP38.3 64.26,51.31 64.26,56.97 v64.95,57.66 | v65.42,67.27 65.42,67.23 65.63,67.01 65.63,66.17 65.89,65.91 67.67,65.91 67.92,66.15 68.38,66.15 68.81,65.72 68.81,65.13 68.57,64.88 68.57,64.2 68.75,64.02 70.44,64.02 70.44,64 70.82,63.62 71.44,63.62 71.54,63.52 71.54,62.76 70.96,62.17 70.27,62.17 69.97,62.47 69.79,62.47 69.64,62.33 69.64,62.11 U20.1 69.65,62.11
  Bottom 0.203: v65.42,67.27 65.39,67.27 64.72,66.61 64.72,64.58 64.26,64.12 64.26,59.82 64.95,59.13 v64.95,57.66
D126
  Top 0.203: JP37.12 78.23,45.64 76.99,46.89 76.99,53.39 75.96,54.41 75.25,54.41 U20.30
D130  (via drill 0.25)
  Top 0.203: R58.1 64.52,46.39 64.52,48.51 64.67,48.67 64.67,55.02 v65.44,55.79 | 67.22,59.66 66.68,60.2 v65.79,60.2
  Bottom 0.203: v65.79,60.2 65.79,56.14 v65.44,55.79
D131  (via drill 0.25)
  Top 0.203: 91.96,55.3 93.27,53.99 94.09,53.99 94.84,53.24 94.84,46.18 95.13,45.9 v95.17,45.9
  Bottom 0.203: JP42.1 82.04,44.2 94.77,44.2 95.17,44.6 v95.17,45.9
D132  (via drill 0.25)
  Top 0.203: U22.28 92.99,53.57 93.81,53.57 94.39,52.99 94.39,46.35 94.4,46.34 v94.4,44.95
  Bottom 0.203: JP42.2 84.15,44.63 94.08,44.63 v94.4,44.95
D133  (via drill 0.25)
  Top 0.203: 86.89,54.25 86.72,54.08 86.72,53.4 v86.46,53.15
  Bottom 0.203: v86.46,53.15 87.63,54.32 87.63,55.12 84.84,57.91 84.84,60.38 84.24,60.97 83.29,60.97 82.94,61.32 82.94,63.91 83.45,64.41 84.16,64.41 84.83,65.08 84.83,67.45 84.84,67.46 84.26,68.04 83.07,68.04 82.56,67.53 82.56,64.73 81.28,63.45 JP42.8
D134  (via drill 0.25)
  Top 0.203: 86.54,54.6 86.03,54.09 v86,54.09
  Bottom 0.203: JP42.7 82.55,58.93 82.55,57.15 83.06,56.64 83.06,55.24 84.21,54.09 v86,54.09
D135  (via drill 0.25)
  Top 0.203: 90.56,53.9 91.61,52.86 v91.61,52.45
  Bottom 0.203: JP42.6 82.55,56.39 82.55,54.41 82.93,54.03 82.93,51.64 83.43,51.14 83.43,48.95 83.9,48.48 88.94,48.48 90.59,50.13 90.59,50.79 91.61,51.81 v91.61,52.45
D136  (via drill 0.25)
  Top 0.203: 92.65,56 93.28,55.36 v93.64,55.36
  Bottom 0.203: JP42.5 82.55,53.85 82.55,52.07 82.51,52.03 82.51,51.45 83,50.95 83,48.76 83.77,47.99 89.06,47.99 91.01,49.93 91.01,50.55 91.02,50.55 91.72,51.24 92.26,51.24 92.87,51.85 92.87,52.38 92.12,53.13 91.14,53.13 90.86,53.42 90.86,54.25 91.42,54.82 93.1,54.82 v93.64,55.36
D137  (via drill 0.25)
  Top 0.203: v91.57,53.98 91.57,54.28 v91.57,53.98 | U22.27 91.57,54.29 v91.57,53.98
  Bottom 0.203: v91.57,53.98 92.02,53.98 93.38,52.61 93.38,51.71 92.5,50.84 91.88,50.84 91.42,50.38 91.42,49.71 89.18,47.47 83.54,47.47 82.52,48.49 82.52,50.76 81.28,52 JP42.4
D138  (via drill 0.25)
  Top 0.203: JP42.3 82.55,51.31 82.55,56.97 v83.24,57.66 | v83.71,67.27 83.71,67.23 83.92,67.01 83.92,66.17 84.18,65.91 85.96,65.91 86.2,66.15 86.67,66.15 87.1,65.72 87.1,65.13 86.86,64.88 86.86,64.2 87.04,64.02 88.72,64.02 88.72,64 89.11,63.62 89.73,63.62 89.83,63.52 89.83,62.76 89.25,62.17 88.56,62.17 88.25,62.47 88.08,62.47 87.93,62.33 87.93,62.11 U22.1 87.94,62.11
  Bottom 0.203: v83.71,67.27 83.67,67.27 83.01,66.61 83.01,64.58 82.55,64.12 82.55,59.82 83.24,59.13 v83.24,57.66
D139
  Top 0.203: JP41.12 96.52,45.64 95.28,46.89 95.28,53.39 94.25,54.41 93.54,54.41 U22.30
D143  (via drill 0.25)
  Top 0.203: R64.1 82.8,46.39 82.8,48.51 82.96,48.67 82.96,55.02 v83.73,55.79 | 85.51,59.66 84.97,60.2 v84.07,60.2
  Bottom 0.203: v84.07,60.2 84.07,56.14 v83.73,55.79
D144  (via drill 0.25)
  Top 0.203: 110.24,55.3 111.56,53.99 112.38,53.99 113.13,53.24 113.13,46.18 113.41,45.9 v113.46,45.9
  Bottom 0.203: JP46.1 100.33,44.2 113.06,44.2 113.46,44.6 v113.46,45.9
D145  (via drill 0.25)
  Top 0.203: U24.28 111.28,53.57 112.1,53.57 112.67,52.99 112.67,46.35 112.69,46.34 v112.69,44.95
  Bottom 0.203: JP46.2 102.44,44.63 112.37,44.63 v112.69,44.95
D146  (via drill 0.25)
  Top 0.203: 105.18,54.25 105,54.08 105,53.4 v104.75,53.15
  Bottom 0.203: v104.75,53.15 105.92,54.32 105.92,55.12 103.12,57.91 103.12,60.38 102.53,60.97 101.58,60.97 101.23,61.32 101.23,63.91 101.74,64.41 102.45,64.41 103.12,65.08 103.12,67.45 103.12,67.46 102.55,68.04 101.35,68.04 100.85,67.53 100.85,64.73 99.57,63.45 JP46.8
D147  (via drill 0.25)
  Top 0.203: 104.83,54.6 104.32,54.09 v104.29,54.09
  Bottom 0.203: JP46.7 100.84,58.93 100.84,57.15 101.35,56.64 101.35,55.24 102.5,54.09 v104.29,54.09
D148  (via drill 0.25)
  Top 0.203: 108.85,53.9 109.9,52.86 v109.9,52.45
  Bottom 0.203: JP46.6 100.84,56.39 100.84,54.41 101.22,54.03 101.22,51.64 101.71,51.14 101.71,48.95 102.19,48.48 107.23,48.48 108.88,50.13 108.88,50.79 109.9,51.81 v109.9,52.45
D149  (via drill 0.25)
  Top 0.203: 110.94,56 111.57,55.36 v111.93,55.36
  Bottom 0.203: JP46.5 100.84,53.85 100.84,52.07 100.8,52.03 100.8,51.45 101.29,50.95 101.29,48.76 102.06,47.99 107.35,47.99 109.3,49.93 109.3,50.55 109.31,50.55 110,51.24 110.55,51.24 111.16,51.85 111.16,52.38 110.41,53.13 109.43,53.13 109.14,53.42 109.14,54.25 109.71,54.82 111.38,54.82 v111.93,55.36
D150  (via drill 0.25)
  Top 0.203: v109.86,53.98 109.86,54.28 v109.86,53.98 | U24.27 109.86,54.29 v109.86,53.98
  Bottom 0.203: v109.86,53.98 110.31,53.98 111.67,52.61 111.67,51.71 110.79,50.84 110.17,50.84 109.71,50.38 109.71,49.71 107.47,47.47 101.83,47.47 100.81,48.49 100.81,50.76 99.57,52 JP46.4
D151  (via drill 0.25)
  Top 0.203: JP46.3 100.84,51.31 100.84,56.97 v101.53,57.66 | v102,67.27 102,67.23 102.21,67.01 102.21,66.17 102.47,65.91 104.24,65.91 104.49,66.15 104.96,66.15 105.39,65.72 105.39,65.13 105.14,64.88 105.14,64.2 105.33,64.02 107.01,64.02 107.01,64 107.39,63.62 108.02,63.62 108.12,63.52 108.12,62.76 107.54,62.17 106.84,62.17 106.54,62.47 106.36,62.47 106.22,62.33 106.22,62.11 U24.1 106.22,62.11
  Bottom 0.203: v102,67.27 101.96,67.27 101.3,66.61 101.3,64.58 100.84,64.12 100.84,59.82 101.53,59.13 v101.53,57.66
D152
  Top 0.203: JP45.12 114.81,45.64 113.56,46.89 113.56,53.39 112.54,54.41 111.83,54.41 U24.30
D156  (via drill 0.25)
  Top 0.203: R70.1 101.09,46.39 101.09,48.51 101.25,48.67 101.25,55.02 v102.01,55.79 | 103.79,59.66 103.25,60.2 v102.36,60.2
  Bottom 0.203: v102.36,60.2 102.36,56.14 v102.01,55.79
D157  (via drill 0.25)
  Top 0.203: 18.8,92.13 20.12,90.82 20.94,90.82 21.69,90.07 21.69,83.01 21.97,82.72 v22.02,82.72
  Bottom 0.203: JP50.1 8.89,81.03 21.61,81.03 22.02,81.43 v22.02,82.72
D158  (via drill 0.25)
  Top 0.203: U26.28 19.84,90.4 20.66,90.4 21.23,89.83 21.23,83.19 21.25,83.17 v21.25,81.78
  Bottom 0.203: JP50.2 11,81.46 20.93,81.46 v21.25,81.78
D159  (via drill 0.25)
  Top 0.203: 13.74,91.08 13.56,90.91 13.56,90.23 v13.31,89.98
  Bottom 0.203: v13.31,89.98 14.48,91.15 14.48,91.95 11.68,94.74 11.68,97.21 11.09,97.8 10.13,97.8 9.79,98.15 9.79,100.74 10.3,101.24 11.01,101.24 11.68,101.92 11.68,104.28 11.68,104.29 11.11,104.87 9.91,104.87 9.41,104.36 9.41,101.56 8.13,100.28 JP50.8
D160  (via drill 0.25)
  Top 0.203: 13.39,91.43 12.88,90.92 v12.85,90.92
  Bottom 0.203: JP50.7 9.4,95.76 9.4,93.98 9.91,93.47 9.91,92.08 11.06,90.92 v12.85,90.92
D161  (via drill 0.25)
  Top 0.203: 17.41,90.73 18.46,89.69 v18.46,89.28
  Bottom 0.203: JP50.6 9.4,93.22 9.4,91.24 9.78,90.86 9.78,88.47 10.27,87.97 10.27,85.78 10.75,85.31 15.79,85.31 17.44,86.97 17.44,87.62 18.46,88.64 v18.46,89.28
D162  (via drill 0.25)
  Top 0.203: 19.5,92.83 20.13,92.19 v20.49,92.19
  Bottom 0.203: JP50.5 9.4,90.68 9.4,88.9 9.36,88.86 9.36,88.28 9.85,87.78 9.85,85.58 10.62,84.82 15.91,84.82 17.86,86.76 17.86,87.38 17.87,87.38 18.57,88.07 19.11,88.07 19.72,88.68 19.72,89.21 18.97,89.96 17.99,89.96 17.7,90.25 17.7,91.08 18.27,91.65 19.94,91.65 v20.49,92.19
D163  (via drill 0.25)
  Top 0.203: v18.41,90.81 18.41,91.11 v18.41,90.81 | U26.27 18.41,91.12 v18.41,90.81
  Bottom 0.203: v18.41,90.81 18.86,90.81 20.23,89.44 20.23,88.54 19.35,87.67 18.73,87.67 18.27,87.21 18.27,86.54 16.03,84.3 10.39,84.3 9.37,85.32 9.37,87.59 8.13,88.83 JP50.4
D164  (via drill 0.25)
  Top 0.203: JP50.3 9.4,88.14 9.4,93.8 v10.09,94.49 | v10.56,104.1 10.56,104.06 10.77,103.84 10.77,103 11.03,102.73 12.8,102.73 13.05,102.98 13.52,102.98 13.95,102.55 13.95,101.96 13.7,101.71 13.7,101.03 13.89,100.85 15.57,100.85 15.57,100.83 15.95,100.45 16.58,100.45 16.68,100.34 16.68,99.59 16.1,99 15.4,99 15.1,99.3 14.93,99.3 14.78,99.16 14.78,98.94 U26.1 14.79,98.94
  Bottom 0.203: v10.56,104.1 10.52,104.1 9.86,103.44 9.86,101.41 9.4,100.95 9.4,96.65 10.09,95.96 v10.09,94.49
D165
  Top 0.203: JP49.12 23.37,82.47 22.12,83.72 22.12,90.22 21.1,91.24 20.39,91.24 U26.30
D169  (via drill 0.25)
  Top 0.203: R76.1 9.65,83.22 9.65,85.34 9.81,85.5 9.81,91.85 v10.57,92.62 | 12.35,96.49 11.81,97.03 v10.92,97.03
  Bottom 0.203: v10.92,97.03 10.92,92.97 v10.57,92.62
D170  (via drill 0.25)
  Top 0.203: 37.09,92.13 38.4,90.82 39.23,90.82 39.98,90.07 39.98,83.01 40.26,82.72 v40.3,82.72
  Bottom 0.203: JP54.1 27.18,81.03 39.9,81.03 40.3,81.43 v40.3,82.72
D171  (via drill 0.25)
  Top 0.203: U28.28 38.13,90.4 38.95,90.4 39.52,89.83 39.52,83.19 39.53,83.17 v39.53,81.78
  Bottom 0.203: JP54.2 29.29,81.46 39.22,81.46 v39.53,81.78
D172  (via drill 0.25)
  Top 0.203: 32.02,91.08 31.85,90.91 31.85,90.23 v31.59,89.98
  Bottom 0.203: v31.59,89.98 32.77,91.15 32.77,91.95 29.97,94.74 29.97,97.21 29.38,97.8 28.42,97.8 28.08,98.15 28.08,100.74 28.59,101.24 29.3,101.24 29.97,101.92 29.97,104.28 29.97,104.29 29.39,104.87 28.2,104.87 27.7,104.36 27.7,101.56 26.42,100.28 JP54.8
D173  (via drill 0.25)
  Top 0.203: 31.68,91.43 31.17,90.92 v31.14,90.92
  Bottom 0.203: JP54.7 27.69,95.76 27.69,93.98 28.19,93.47 28.19,92.08 29.34,90.92 v31.14,90.92
D174  (via drill 0.25)
  Top 0.203: 35.7,90.73 36.74,89.69 v36.74,89.28
  Bottom 0.203: JP54.6 27.69,93.22 27.69,91.24 28.07,90.86 28.07,88.47 28.56,87.97 28.56,85.78 29.04,85.31 34.07,85.31 35.73,86.97 35.73,87.62 36.74,88.64 v36.74,89.28
D175  (via drill 0.25)
  Top 0.203: 37.79,92.83 38.42,92.19 v38.78,92.19
  Bottom 0.203: JP54.5 27.69,90.68 27.69,88.9 27.64,88.86 27.64,88.28 28.14,87.78 28.14,85.58 28.91,84.82 34.2,84.82 36.14,86.76 36.14,87.38 36.16,87.38 36.85,88.07 37.4,88.07 38.01,88.68 38.01,89.21 37.26,89.96 36.28,89.96 35.99,90.25 35.99,91.08 36.56,91.65 38.23,91.65 v38.78,92.19
D176  (via drill 0.25)
  Top 0.203: v36.7,90.81 36.7,91.11 v36.7,90.81 | U28.27 36.7,91.12 v36.7,90.81
  Bottom 0.203: v36.7,90.81 37.15,90.81 38.52,89.44 38.52,88.54 37.64,87.67 37.02,87.67 36.56,87.21 36.56,86.54 34.31,84.3 28.68,84.3 27.66,85.32 27.66,87.59 26.42,88.83 JP54.4
D177  (via drill 0.25)
  Top 0.203: JP54.3 27.69,88.14 27.69,93.8 v28.38,94.49 | v28.84,104.1 28.84,104.06 29.06,103.84 29.06,103 29.32,102.73 31.09,102.73 31.34,102.98 31.81,102.98 32.23,102.55 32.23,101.96 31.99,101.71 31.99,101.03 32.17,100.85 33.86,100.85 33.86,100.83 34.24,100.45 34.86,100.45 34.97,100.34 34.97,99.59 34.38,99 33.69,99 33.39,99.3 33.21,99.3 33.07,99.16 33.07,98.94 U28.1 33.07,98.94
  Bottom 0.203: v28.84,104.1 28.81,104.1 28.14,103.44 28.14,101.41 27.69,100.95 27.69,96.65 28.38,95.96 v28.38,94.49
D178
  Top 0.203: JP53.12 41.66,82.47 40.41,83.72 40.41,90.22 39.38,91.24 38.67,91.24 U28.30
D182  (via drill 0.25)
  Top 0.203: R82.1 27.94,83.22 27.94,85.34 28.09,85.5 28.09,91.85 v28.86,92.62 | 30.64,96.49 30.1,97.03 v29.21,97.03
  Bottom 0.203: v29.21,97.03 29.21,92.97 v28.86,92.62
D183  (via drill 0.25)
  Top 0.203: 55.38,92.13 56.69,90.82 57.52,90.82 58.27,90.07 58.27,83.01 58.55,82.72 v58.59,82.72
  Bottom 0.203: JP58.1 45.47,81.03 58.19,81.03 58.59,81.43 v58.59,82.72
D184  (via drill 0.25)
  Top 0.203: U30.28 56.42,90.4 57.24,90.4 57.81,89.83 57.81,83.19 57.82,83.17 v57.82,81.78
  Bottom 0.203: JP58.2 47.57,81.46 57.5,81.46 v57.82,81.78
D185  (via drill 0.25)
  Top 0.203: 50.31,91.08 50.14,90.91 50.14,90.23 v49.88,89.98
  Bottom 0.203: v49.88,89.98 51.05,91.15 51.05,91.95 48.26,94.74 48.26,97.21 47.67,97.8 46.71,97.8 46.37,98.15 46.37,100.74 46.88,101.24 47.59,101.24 48.26,101.92 48.26,104.28 48.26,104.29 47.68,104.87 46.49,104.87 45.99,104.36 45.99,101.56 44.7,100.28 JP58.8
D186  (via drill 0.25)
  Top 0.203: 49.97,91.43 49.96,91.43 49.46,90.92 v49.42,90.92
  Bottom 0.203: JP58.7 45.97,95.76 45.97,93.98 46.48,93.47 46.48,92.08 47.63,90.92 v49.42,90.92
D187  (via drill 0.25)
  Top 0.203: 53.99,90.73 55.03,89.69 v55.03,89.28
  Bottom 0.203: JP58.6 45.97,93.22 45.97,91.24 46.35,90.86 46.35,88.47 46.85,87.97 46.85,85.78 47.33,85.31 52.36,85.31 54.02,86.97 54.02,87.62 55.03,88.64 v55.03,89.28
D188  (via drill 0.25)
  Top 0.203: 56.08,92.83 56.71,92.19 v57.06,92.19
  Bottom 0.203: JP58.5 45.97,90.68 45.97,88.9 45.93,88.86 45.93,88.28 46.43,87.78 46.43,85.58 47.19,84.82 52.49,84.82 54.43,86.76 54.43,87.38 54.45,87.38 55.14,88.07 55.68,88.07 56.29,88.68 56.29,89.21 55.55,89.96 54.56,89.96 54.28,90.25 54.28,91.08 54.85,91.65 56.52,91.65 v57.06,92.19
D189  (via drill 0.25)
  Top 0.203: v54.99,90.81 54.99,91.11 v54.99,90.81 | U30.27 54.99,91.12 v54.99,90.81
  Bottom 0.203: v54.99,90.81 55.44,90.81 56.81,89.44 56.81,88.54 55.93,87.67 55.31,87.67 54.85,87.21 54.85,86.54 52.6,84.3 46.97,84.3 45.95,85.32 45.95,87.59 44.7,88.83 JP58.4
D190  (via drill 0.25)
  Top 0.203: JP58.3 45.97,88.14 45.97,93.8 v46.66,94.49 | v47.13,104.1 47.13,104.06 47.35,103.84 47.35,103 47.61,102.73 49.38,102.73 49.63,102.98 50.09,102.98 50.52,102.55 50.52,101.96 50.28,101.71 50.28,101.03 50.46,100.85 52.15,100.85 52.15,100.83 52.53,100.45 53.15,100.45 53.25,100.34 53.25,99.59 52.67,99 51.98,99 51.68,99.3 51.5,99.3 51.35,99.16 51.35,98.94 U30.1 51.36,98.94
  Bottom 0.203: v47.13,104.1 47.1,104.1 46.43,103.44 46.43,101.41 45.97,100.95 45.97,96.65 46.66,95.96 v46.66,94.49
D191
  Top 0.203: JP57.12 59.94,82.47 58.7,83.72 58.7,90.22 57.67,91.24 56.96,91.24 U30.30
D195  (via drill 0.25)
  Top 0.203: R88.1 46.23,83.22 46.23,85.34 46.38,85.5 46.38,91.85 v47.15,92.62 | 48.93,96.49 48.39,97.03 v47.5,97.03
  Bottom 0.203: v47.5,97.03 47.5,92.97 v47.15,92.62
D196  (via drill 0.25)
  Top 0.203: 73.67,92.13 74.98,90.82 75.81,90.82 76.56,90.07 76.56,83.01 76.84,82.72 v76.88,82.72
  Bottom 0.203: JP62.1 63.75,81.03 76.48,81.03 76.88,81.43 v76.88,82.72
D197  (via drill 0.25)
  Top 0.203: U32.28 74.7,90.4 75.53,90.4 76.1,89.83 76.1,83.19 76.11,83.17 v76.11,81.78
  Bottom 0.203: JP62.2 65.86,81.46 75.79,81.46 v76.11,81.78
D198  (via drill 0.25)
  Top 0.203: 68.6,91.08 68.43,90.91 68.43,90.23 v68.17,89.98
  Bottom 0.203: v68.17,89.98 69.34,91.15 69.34,91.95 66.55,94.74 66.55,97.21 65.96,97.8 65,97.8 64.66,98.15 64.66,100.74 65.16,101.24 65.88,101.24 66.55,101.92 66.55,104.28 66.55,104.29 65.97,104.87 64.78,104.87 64.28,104.36 64.28,101.56 62.99,100.28 JP62.8
D199  (via drill 0.25)
  Top 0.203: 68.25,91.43 67.74,90.92 v67.71,90.92
  Bottom 0.203: JP62.7 64.26,95.76 64.26,93.98 64.77,93.47 64.77,92.08 65.92,90.92 v67.71,90.92
D200  (via drill 0.25)
  Top 0.203: 72.27,90.73 73.32,89.69 v73.32,89.28
  Bottom 0.203: JP62.6 64.26,93.22 64.26,91.24 64.64,90.86 64.64,88.47 65.14,87.97 65.14,85.78 65.61,85.31 70.65,85.31 72.31,86.97 72.31,87.62 73.32,88.64 v73.32,89.28
D201  (via drill 0.25)
  Top 0.203: 74.37,92.83 75,92.19 v75.35,92.19
  Bottom 0.203: JP62.5 64.26,90.68 64.26,88.9 64.22,88.86 64.22,88.28 64.72,87.78 64.72,85.58 65.48,84.82 70.78,84.82 72.72,86.76 72.72,87.38 72.73,87.38 73.43,88.07 73.97,88.07 74.58,88.68 74.58,89.21 73.83,89.96 72.85,89.96 72.57,90.25 72.57,91.08 73.13,91.65 74.81,91.65 v75.35,92.19
D202  (via drill 0.25)
  Top 0.203: v73.28,90.81 73.28,91.11 v73.28,90.81 | U32.27 73.28,91.12 v73.28,90.81
  Bottom 0.203: v73.28,90.81 73.73,90.81 75.09,89.44 75.09,88.54 74.22,87.67 73.59,87.67 73.13,87.21 73.13,86.54 70.89,84.3 65.25,84.3 64.23,85.32 64.23,87.59 62.99,88.83 JP62.4
D203  (via drill 0.25)
  Top 0.203: JP62.3 64.26,88.14 64.26,93.8 v64.95,94.49 | v65.42,104.1 65.42,104.06 65.63,103.84 65.63,103 65.89,102.73 67.67,102.73 67.92,102.98 68.38,102.98 68.81,102.55 68.81,101.96 68.57,101.71 68.57,101.03 68.75,100.85 70.44,100.85 70.44,100.83 70.82,100.45 71.44,100.45 71.54,100.34 71.54,99.59 70.96,99 70.27,99 69.97,99.3 69.79,99.3 69.64,99.16 69.64,98.94 U32.1 69.65,98.94
  Bottom 0.203: v65.42,104.1 65.39,104.1 64.72,103.44 64.72,101.41 64.26,100.95 64.26,96.65 64.95,95.96 v64.95,94.49
D204
  Top 0.203: JP61.12 78.23,82.47 76.99,83.72 76.99,90.22 75.96,91.24 75.25,91.24 U32.30
D208  (via drill 0.25)
  Top 0.203: R94.1 64.52,83.22 64.52,85.34 64.67,85.5 64.67,91.85 v65.44,92.62 | 67.22,96.49 66.68,97.03 v65.79,97.03
  Bottom 0.203: v65.79,97.03 65.79,92.97 v65.44,92.62
D209  (via drill 0.25)
  Top 0.203: 91.96,92.13 93.27,90.82 94.09,90.82 94.84,90.07 94.84,83.01 95.13,82.72 v95.17,82.72
  Bottom 0.203: JP66.1 82.04,81.03 94.77,81.03 95.17,81.43 v95.17,82.72
D210  (via drill 0.25)
  Top 0.203: U34.28 92.99,90.4 93.81,90.4 94.39,89.83 94.39,83.19 94.4,83.17 v94.4,81.78
  Bottom 0.203: JP66.2 84.15,81.46 94.08,81.46 v94.4,81.78
D211  (via drill 0.25)
  Top 0.203: 86.89,91.08 86.72,90.91 86.72,90.23 v86.46,89.98
  Bottom 0.203: v86.46,89.98 87.63,91.15 87.63,91.95 84.84,94.74 84.84,97.21 84.24,97.8 83.29,97.8 82.94,98.15 82.94,100.74 83.45,101.24 84.16,101.24 84.83,101.92 84.83,104.28 84.84,104.29 84.26,104.87 83.07,104.87 82.56,104.36 82.56,101.56 81.28,100.28 JP66.8
D212  (via drill 0.25)
  Top 0.203: 86.54,91.43 86.03,90.92 v86,90.92
  Bottom 0.203: JP66.7 82.55,95.76 82.55,93.98 83.06,93.47 83.06,92.08 84.21,90.92 v86,90.92
D213  (via drill 0.25)
  Top 0.203: 90.56,90.73 91.61,89.69 v91.61,89.28
  Bottom 0.203: JP66.6 82.55,93.22 82.55,91.24 82.93,90.86 82.93,88.47 83.43,87.97 83.43,85.78 83.9,85.31 88.94,85.31 90.59,86.97 90.59,87.62 91.61,88.64 v91.61,89.28
D214  (via drill 0.25)
  Top 0.203: 92.65,92.83 93.28,92.19 v93.64,92.19
  Bottom 0.203: JP66.5 82.55,90.68 82.55,88.9 82.51,88.86 82.51,88.28 83,87.78 83,85.58 83.77,84.82 89.06,84.82 91.01,86.76 91.01,87.38 91.02,87.38 91.72,88.07 92.26,88.07 92.87,88.68 92.87,89.21 92.12,89.96 91.14,89.96 90.86,90.25 90.86,91.08 91.42,91.65 93.1,91.65 v93.64,92.19
D215  (via drill 0.25)
  Top 0.203: v91.57,90.81 91.57,91.11 v91.57,90.81 | U34.27 91.57,91.12 v91.57,90.81
  Bottom 0.203: v91.57,90.81 92.02,90.81 93.38,89.44 93.38,88.54 92.5,87.67 91.88,87.67 91.42,87.21 91.42,86.54 89.18,84.3 83.54,84.3 82.52,85.32 82.52,87.59 81.28,88.83 JP66.4
D216  (via drill 0.25)
  Top 0.203: JP66.3 82.55,88.14 82.55,93.8 v83.24,94.49 | v83.71,104.1 83.71,104.06 83.92,103.84 83.92,103 84.18,102.73 85.96,102.73 86.2,102.98 86.67,102.98 87.1,102.55 87.1,101.96 86.86,101.71 86.86,101.03 87.04,100.85 88.72,100.85 88.72,100.83 89.11,100.45 89.73,100.45 89.83,100.34 89.83,99.59 89.25,99 88.56,99 88.25,99.3 88.08,99.3 87.93,99.16 87.93,98.94 U34.1 87.94,98.94
  Bottom 0.203: v83.71,104.1 83.67,104.1 83.01,103.44 83.01,101.41 82.55,100.95 82.55,96.65 83.24,95.96 v83.24,94.49
D217
  Top 0.203: JP65.12 96.52,82.47 95.28,83.72 95.28,90.22 94.25,91.24 93.54,91.24 U34.30
D221  (via drill 0.25)
  Top 0.203: R100.1 82.8,83.22 82.8,85.34 82.96,85.5 82.96,91.85 v83.73,92.62 | 85.51,96.49 84.97,97.03 v84.07,97.03
  Bottom 0.203: v84.07,97.03 84.07,92.97 v83.73,92.62
D222  (via drill 0.25)
  Top 0.203: 110.24,92.13 111.56,90.82 112.38,90.82 113.13,90.07 113.13,83.01 113.41,82.72 v113.46,82.72
  Bottom 0.203: JP70.1 100.33,81.03 113.06,81.03 113.46,81.43 v113.46,82.72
